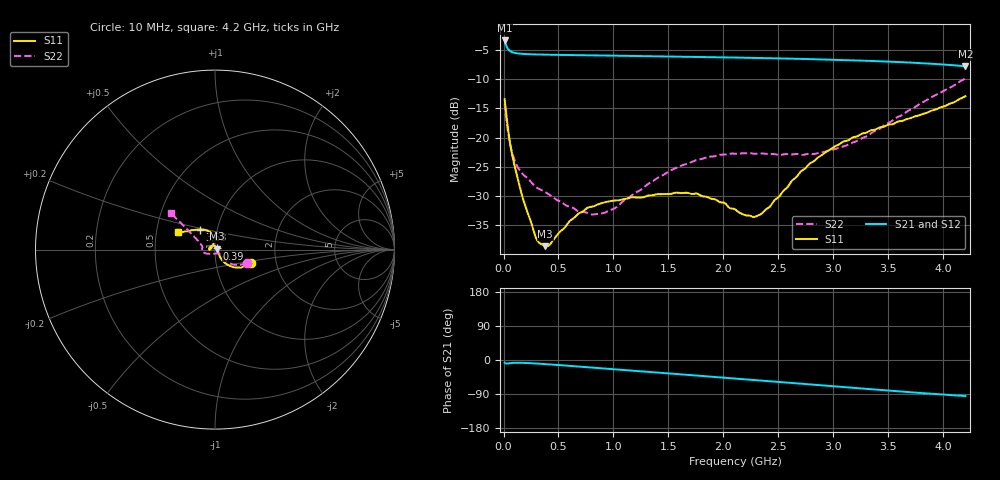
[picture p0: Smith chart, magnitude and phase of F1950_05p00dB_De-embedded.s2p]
! Integrated Device Technology
! Corporate Headquarters
! 6024 Silver Creek Valley Road
! San Jose, CA 95138  USA
! Phone:  1-408-284-8200
! Toll Free:  1-800-223-1366
! Webpage:  http://www.idt.com/
! Timing and RF Division
! 515 Groton Road, Suite 102
! Westford, MA 01886-6024
! Device:  F1950
! Description: 7-bit 0.25 dB Digital Step Attenuator
! Frequency:  150.0 -  4000.00 MHz
! Package:  4x4 mm Thin QFN Plastic Package: 24 pin
! Ports:  2 RF, 12 DC
!  Pin  1  = D0
!  Pin  2  = VDD
!  Pin  3  = Vmode
!  Pin  4  = GND
!  Pin  5  = RF1  =  Port 1
!  Pin  6  = GND
!  Pin  7  = GND
!  Pin  8  = GND
!  Pin  9  = GND
!  Pin 10  = GND
!  Pin 11  = GND
!  Pin 12  = GND
!  Pin 13  = GND
!  Pin 14  = RF2  =  Port 2
!  Pin 15  = GND
!  Pin 16  = LE
!  Pin 17  = CLK
!  Pin 18  = DATE
!  Pin 19  = D6
!  Pin 20  = D5
!  Pin 21  = D4
!  Pin 22  = D3
!  Pin 23  = D2
!  Pin 24  = D1
! State:  20
! Atten State:  5.00 dB
! Voltage:  +5.00 Volts
! Current:  Not Measured mA
! Data:  The device was measured on a the F195X evaluation board which has
!  individual transmission lines to the RF pins.  Data was collected
!  using a calibrated network analyzer.  The evaluation board was
!  de-embedded using a TRL calibration technique.
!  The reference plane is the edge of the package pin.
! Misc:  Board 2019
!  Action Tracker AT0250
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# GHz S dB R 50
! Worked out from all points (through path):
!   420 points, 10 MHz to 4.2 GHz, reference 50 ohm
!   highest |S21| = -3.41 dB at 10 MHz (marker M1); lowest = -7.8 dB at 4.2 GHz (marker M2)
!   group delay of S21, straight-line fit = 61.5 ps
!   lowest |S11| = -38.5 dB at 380 MHz (marker M3), VSWR 1.02, Z = 51.1 + j0.561 ohm
!   |S11| at or under -10 dB: start of sweep to end of sweep
!   |S22| runs from -33.1 to -9.9 dB; largest |S21 - S12| = 0.00051
!   S11 on the Smith chart (normalised r, x): 10 MHz: 1.47, -0.24; 390 MHz: 1.02, +0.01; 3.63 GHz: 0.83, +0.19; 4.2 GHz: 0.65, +0.13
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0.01  -13.43 -21.0  -3.41 -7.1  -3.41 -7.1  -14.21 -23.3
0.04  -18.36 -48.1  -4.85 -9.2  -4.85 -9.2  -18.95 -42.6
0.07  -22.09 -55.1  -5.34 -8.0  -5.34 -8.0  -21.88 -44.0
0.12  -26.28 -55.2  -5.60 -7.2  -5.60 -7.2  -24.71 -40.4
0.18  -30.62 -44.4  -5.71 -7.5  -5.71 -7.5  -26.33 -41.6
0.29  -36.87 -13.0  -5.80 -9.1  -5.80 -9.1  -28.38 -42.2
0.33  -38.05 3.0  -5.82 -9.9  -5.82 -9.9  -28.80 -43.5
0.38  -38.53 27.6  -5.84 -10.8  -5.84 -10.8  -29.32 -44.1
0.39  -38.52 32.5  -5.84 -11.0  -5.84 -11.0  -29.44 -44.1
0.71  -32.72 103.9  -5.93 -17.8  -5.93 -17.8  -32.72 -67.0
0.83  -31.65 114.7  -5.96 -20.4  -5.96 -20.4  -33.10 -83.8
1  -30.75 129.0  -6.01 -24.2  -6.01 -24.2  -32.18 -109.8
1.41  -29.65 163.2  -6.12 -33.3  -6.12 -33.3  -26.79 -149.6
1.76  -29.57 -179.6  -6.22 -41.2  -6.22 -41.1  -23.80 -164.7
2.11  -32.29 171.6  -6.34 -49.1  -6.33 -49.1  -22.75 -175.2
2.27  -33.53 146.0  -6.39 -52.7  -6.39 -52.7  -22.73 -179.0
2.34  -33.08 133.1  -6.42 -54.3  -6.42 -54.2  -22.69 179.1
2.81  -24.17 96.7  -6.61 -64.9  -6.60 -64.9  -22.80 166.5
3.12  -20.56 104.1  -6.77 -72.0  -6.76 -72.1  -21.32 158.5
3.51  -17.75 121.0  -7.03 -80.9  -7.02 -80.9  -17.43 148.6
3.63  -17.11 126.9  -7.12 -83.5  -7.12 -83.6  -16.06 146.3
4.2  -12.93 155.0  -7.83 -95.1  -7.83 -95.1  -9.91 140.3
